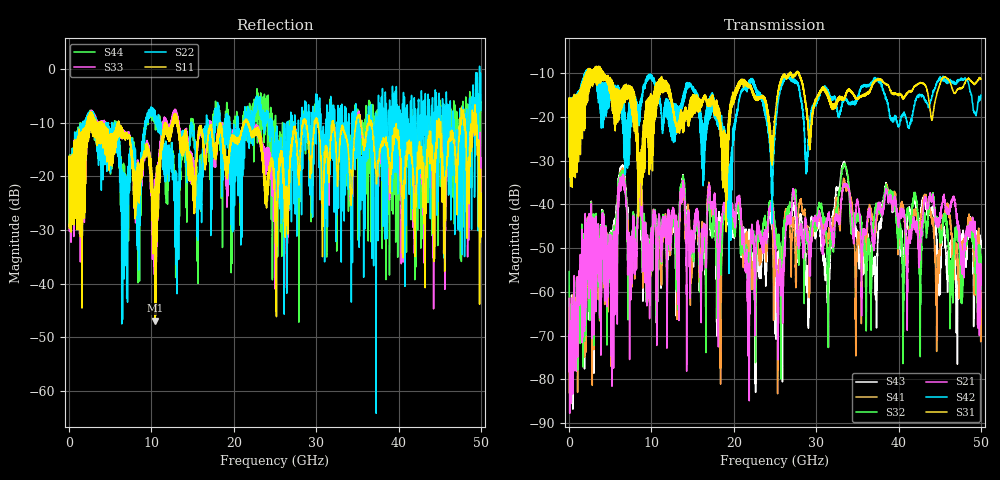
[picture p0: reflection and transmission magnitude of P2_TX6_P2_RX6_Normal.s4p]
!Keysight Technologies,N5225B,MY57041031,A.13.20.10
!Date: Friday, May 31, 2019 11:36:21
!Correction: S11(Full 4 Port(1,2,3,4))
!S12(Full 4 Port(1,2,3,4))
!S13(Full 4 Port(1,2,3,4))
!S14(Full 4 Port(1,2,3,4))
!S21(Full 4 Port(1,2,3,4))
!S22(Full 4 Port(1,2,3,4))
!S23(Full 4 Port(1,2,3,4))
!S24(Full 4 Port(1,2,3,4))
!S31(Full 4 Port(1,2,3,4))
!S32(Full 4 Port(1,2,3,4))
!S33(Full 4 Port(1,2,3,4))
!S34(Full 4 Port(1,2,3,4))
!S41(Full 4 Port(1,2,3,4))
!S42(Full 4 Port(1,2,3,4))
!S43(Full 4 Port(1,2,3,4))
!S44(Full 4 Port(1,2,3,4))
!S4P File: Measurements: <S11,S12,S13,S14>,
!<S21,S22,S23,S24>,
!<S31,S32,S33,S34>,
!<S41,S42,S43,S44>:
# Hz S  dB  R 50.0
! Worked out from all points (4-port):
!   5000 points, 10 MHz to 50 GHz, reference 50 ohm
!   strongest paths, dB at 10 MHz, 12.51 GHz, 25.01 GHz, 37.51 GHz, 50 GHz:
!     S31: -19.3, -16.8, -20.0, -11.6, -11.4
!     S42: -19.3, -16.9, -23.6, -11.2, -15.1
!     S21: -61.5, -42.9, -50.0, -40.6, -56.2
!     S32: -55.4, -44.0, -44.9, -40.3, -53.3
!     S41: -72.5, -43.8, -53.1, -41.5, -66.9
!     S43: -63.7, -45.5, -59.7, -47.6, -48.3
!   lowest |S11| = -46.9 dB at 10.41 GHz (marker M1), VSWR 1.01, Z = 50 - j0.453 ohm
!   |S11| at or under -10 dB: 13.21 GHz to 21.18 GHz (7.966 GHz wide, 46.3 % of centre); 21.74 GHz to 28.38 GHz (6.638 GHz wide, 26.5 % of centre); 36.76 GHz to 44.63 GHz (7.872 GHz wide, 19.3 % of centre)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
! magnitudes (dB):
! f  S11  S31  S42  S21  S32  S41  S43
! 10 MHz  -19.4  -19.3  -19.3  -61.5  -55.4  -72.5  -63.7
! 6.38 GHz  -12.1  -15.4  -17.4  -33.7  -32.4  -32.2  -31.2
! 10.41 GHz  -46.9  -14.8  -13.3  -41.5  -41.2  -41.4  -41.3
! 19.46 GHz  -15.7  -19.0  -32.5  -39.7  -41.1  -41.8  -43.2
! 22.07 GHz  -11.9  -13.2  -11.5  -48.0  -51.8  -53.0  -52.1
! 38.56 GHz  -14.1  -12.7  -16.4  -36.6  -36.4  -35.4  -35.6
! 50 GHz  -23.2  -11.4  -15.1  -56.2  -53.3  -66.9  -48.3
